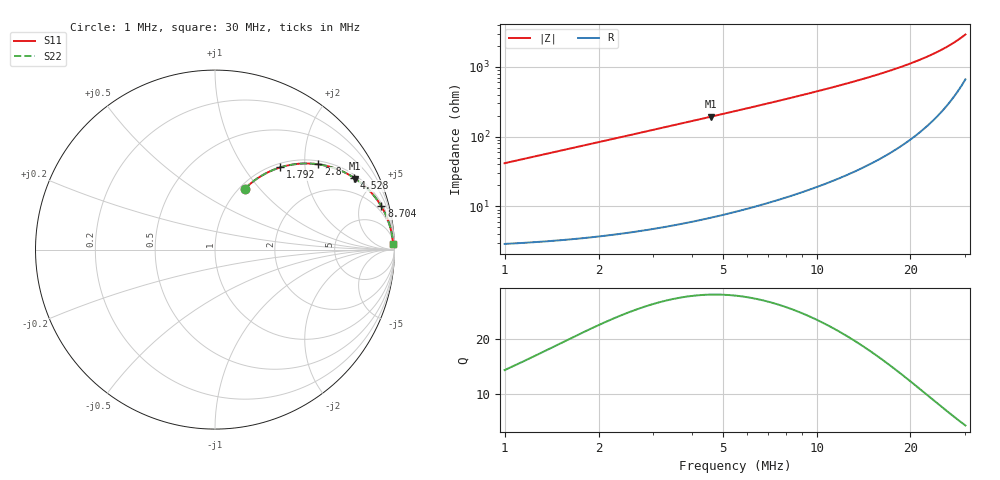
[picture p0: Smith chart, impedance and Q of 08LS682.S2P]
! Coilcraft 0805LS-682 Chip Inductor
! 18 September 2002
# MHZ S MA R 50
!Freq  MagS11  AngS11  MagS21  AngS21  MagS12  AngS12  MagS22  AngS22
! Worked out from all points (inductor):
!   404 points, 1 MHz to 30 MHz, reference 50 ohm
!   read as one part in series: L = 6.63 uH near 1.144 MHz
!   highest Q = 28 at 4.6 MHz (marker M1), where L = 6.71 uH
!   S11 on the Smith chart (normalised r, x): 1 MHz: 1.06, +0.83; 1.792 MHz: 1.07, +1.49; 2.8 MHz: 1.09, +2.34; 4.528 MHz: 1.14, +3.82; 8.704 MHz: 1.31, +7.61; 30 MHz: 14, +57
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1  0.3758 64.0  0.9009 -22.0  0.9009 -22.0  0.3758 64.0
1.144  0.4205 61.6  0.8812 -24.8  0.8812 -24.8  0.4205 61.6
1.432  0.501 56.9  0.8389 -30.0  0.8389 -30.0  0.501 56.9
1.792  0.5857 51.5  0.7834 -35.8  0.7834 -35.8  0.5857 51.5
2.224  0.6666 45.8  0.7178 -41.8  0.7178 -41.8  0.6666 45.8
2.8  0.7463 39.6  0.6373 -48.2  0.6373 -48.2  0.7463 39.6
3.16  0.7838 36.3  0.5923 -51.6  0.5923 -51.6  0.7838 36.3
3.592  0.8196 32.9  0.5438 -55.0  0.5438 -55.0  0.8196 32.9
4.024  0.8476 30.0  0.501 -57.9  0.501 -57.9  0.8476 30.0
4.528  0.8731 27.2  0.4573 -60.8  0.4573 -60.8  0.8731 27.2
4.6  0.8762 26.8  0.4516 -61.1  0.4516 -61.1  0.8762 26.8
5.176  0.8977 24.2  0.4097 -63.8  0.4097 -63.8  0.8977 24.2
5.896  0.9176 21.4  0.3657 -66.5  0.3657 -66.5  0.9176 21.4
7.12  0.9402 17.9  0.3071 -70.0  0.3071 -70.0  0.9402 17.9
8.704  0.9578 14.6  0.2516 -73.1  0.2516 -73.1  0.9578 14.6
10.72  0.9706 11.6  0.2015 -75.9  0.2015 -75.9  0.9706 11.6
12.952  0.9787 9.3  0.162 -77.8  0.162 -77.8  0.9787 9.3
15.544  0.9842 7.4  0.1285 -79.3  0.1285 -79.3  0.9842 7.4
20.368  0.9892 4.9  0.08558 -80.3  0.08558 -80.3  0.9892 4.9
25.192  0.9912 3.2  0.0561 -79.4  0.0561 -79.4  0.9912 3.2
27.568  0.9916 2.5  0.04448 -77.8  0.04448 -77.8  0.9916 2.5
30  0.9917 1.9  0.03402 -75.0  0.03402 -75.0  0.9917 1.9
